(* Logix 5000 DataType export PacketPower_PowerMonitor; software revision 33.00 *)

TYPE PacketPower_PowerMonitor :
STRUCT
   Status : DINT; {access Read Only}   // Power node #1: status mask [1 indicates presence: B0:node, B1:L1, B2:L2, B3:L3]
   DataAge : DINT; {access Read Only}   // Data age [s]
   TotalPower : REAL; {access Read Only}   // Total power [W]
   TotalEnergyLowWord : DINT; {access Read Only}   // Total energy low word [Wh]
   TotalEnergyHighWord : DINT; {access Read Only}   // Total energy high word [Wh]
   LineReadings : PacketPower_SubUDT_PowerLineReading[3];
END_STRUCT
END_TYPE

TYPE PacketPower_SubUDT_PowerLineReading :   // Readings from a single line on a potentially multi-line circuit
STRUCT
   Voltage : REAL; {access Read Only}   // voltage [V]
   Current : REAL; {access Read Only}   // current [A]
   Power : REAL; {access Read Only}   // power [W]
   PowerFactor : REAL; {access Read Only}   // power factor [1]
   Temperature : REAL; {access Read Only}   // temperature [Cel]
END_STRUCT
END_TYPE
